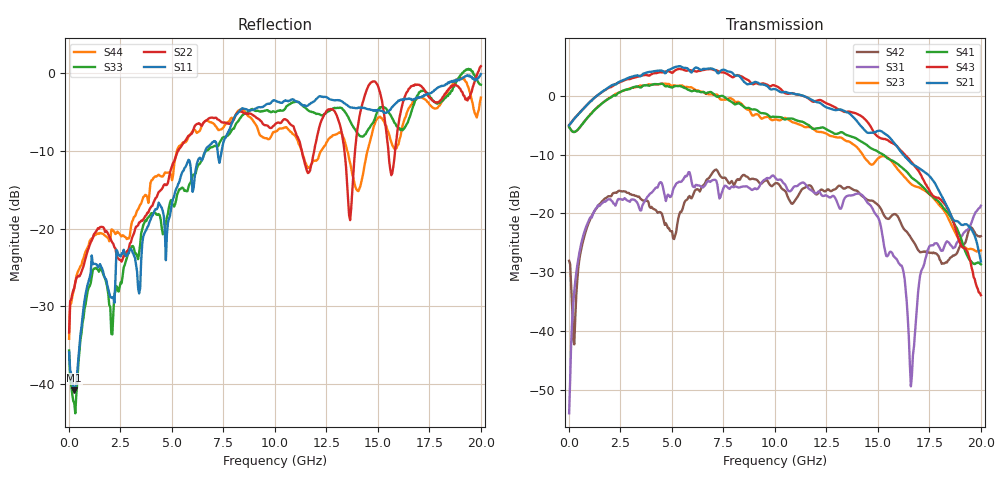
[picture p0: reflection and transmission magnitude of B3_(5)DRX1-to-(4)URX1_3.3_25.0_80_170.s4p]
!Agilent Technologies,N5225A,MY51451112,A.09.50.13
!Agilent N5225A: A.09.50.13
!Date: Sunday, March 12, 2017 05:22:30
!Correction: S11(Full 4 Port(1,2,3,4))
!S12(Full 4 Port(1,2,3,4))
!S13(Full 4 Port(1,2,3,4))
!S14(Full 4 Port(1,2,3,4))
!S21(Full 4 Port(1,2,3,4))
!S22(Full 4 Port(1,2,3,4))
!S23(Full 4 Port(1,2,3,4))
!S24(Full 4 Port(1,2,3,4))
!S31(Full 4 Port(1,2,3,4))
!S32(Full 4 Port(1,2,3,4))
!S33(Full 4 Port(1,2,3,4))
!S34(Full 4 Port(1,2,3,4))
!S41(Full 4 Port(1,2,3,4))
!S42(Full 4 Port(1,2,3,4))
!S43(Full 4 Port(1,2,3,4))
!S44(Full 4 Port(1,2,3,4))
!S4P File: Measurements: <S11,S12,S13,S14>,
!<S21,S22,S23,S24>,
!<S31,S32,S33,S34>,
!<S41,S42,S43,S44>:
# Hz S  dB  R 50
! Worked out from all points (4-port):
!   401 points, 10 MHz to 20 GHz, reference 50 ohm
!   strongest paths, dB at 10 MHz, 5.008 GHz, 10.01 GHz, 15 GHz, 20 GHz:
!     S21: -5.0, 4.6, 1.1, -6.0, -28.2
!     S43: -5.0, 3.9, 1.7, -7.0, -33.9
!     S41: -5.3, 1.4, -3.6, -9.5, -28.7
!     S23: -5.3, 1.7, -4.0, -10.7, -26.3
!     S31: -54.0, -16.8, -13.9, -20.6, -18.7
!     S42: -28.1, -23.0, -14.9, -18.5, -23.9
!   lowest |S11| = -40.8 dB at 259.9 MHz (marker M1), VSWR 1.02, Z = 50.3 - j0.876 ohm
!   |S11| at or under -10 dB: start of sweep to 6.628 GHz; 7.216 GHz to 7.418 GHz (201.9 MHz wide, 2.76 % of centre)
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1e7  -35.90 -39.3  -66.41 109.3  -52.05 18.4  -65.93 46.5
     -5.01 1.8  -33.32 39.7  -5.33 -179.6  -27.97 38.2
     -53.98 17.5  -66.81 144.6  -35.65 -47.4  -75.51 157.7
     -5.33 -179.6  -28.06 38.4  -4.99 1.9  -34.14 44.9
2.59875e8  -40.77 -72.1  -49.87 56.4  -33.13 94.9  -50.38 53.3
           -3.90 3.1  -27.61 -132.0  -6.17 176.8  -41.97 -161.5
           -33.24 95.5  -49.96 58.7  -42.40 -79.5  -50.71 56.0
           -6.17 176.0  -42.26 -170.6  -3.89 2.4  -27.69 -137.8
3.0085e9  -22.67 142.3  -43.76 -15.8  -17.76 51.9  -44.18 -26.3
          3.17 -95.6  -21.77 159.5  1.30 75.6  -16.79 38.4
          -17.70 53.6  -42.61 -8.1  -22.51 117.9  -43.07 -21.0
          1.26 66.3  -16.75 38.5  2.88 -103.0  -19.83 142.4
5.057475e9  -16.18 90.8  -41.11 10.4  -15.95 28.4  -39.23 -28.6
            4.73 172.0  -11.57 146.6  1.75 -24.5  -24.38 44.3
            -15.99 28.4  -37.70 -2.6  -16.98 102.7  -33.27 -40.7
            1.46 -39.6  -24.23 41.6  3.95 161.3  -13.14 126.6
8.2059e9  -5.17 36.5  -38.87 -114.1  -15.67 1.6  -36.78 -141.9
          3.43 15.7  -5.07 82.1  -1.03 -171.0  -13.86 47.4
          -15.59 0.9  -32.78 -112.9  -6.26 59.1  -32.01 -145.0
          -1.34 165.8  -14.18 51.3  3.48 2.8  -4.89 46.1
1.155422e10  -4.26 -6.2  -37.44 -117.7  -14.92 -22.4  -40.09 -136.7
             -0.28 -129.2  -12.59 85.5  -5.33 47.0  -15.33 37.1
             -15.41 -23.6  -33.57 -123.2  -4.69 10.4  -34.11 -152.2
             -4.86 8.8  -15.38 42.1  -0.30 -154.4  -11.91 25.4
2e10  -0.18 -114.1  -32.98 62.9  -18.71 121.3  -35.50 21.1
      -28.18 -159.2  0.84 17.1  -26.30 24.1  -23.89 101.9
      -18.70 121.3  -34.00 40.3  -1.53 -87.7  -35.27 -7.6
      -28.66 -22.8  -23.88 102.8  -33.89 172.5  -3.18 -136.6
